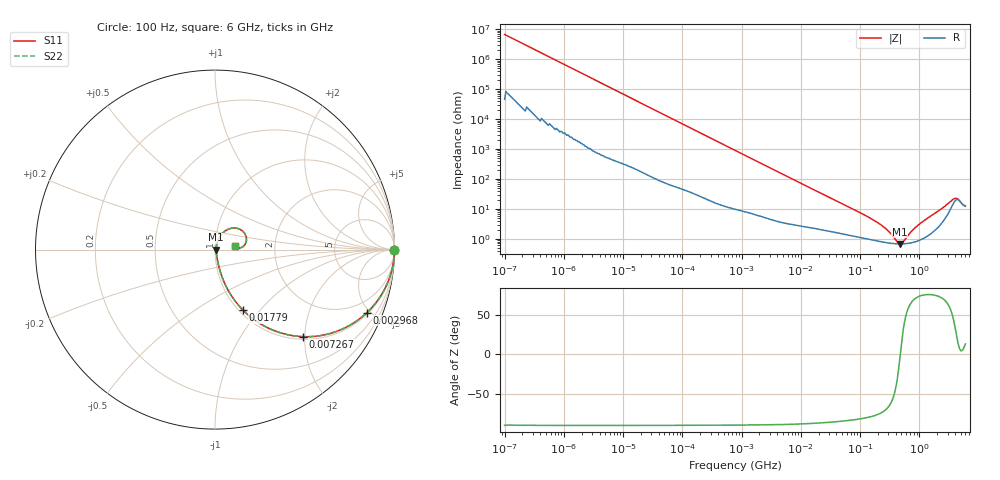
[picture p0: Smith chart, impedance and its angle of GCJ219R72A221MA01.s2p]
!Murata Part Number: GCJ219R72A221MA01
!These Parameters are Measured in Series Mode Connection
!Data Generated on Mar 13, 2026
!  o--ll--o
!Port1  Port2
!  o------o
!Operation Temp=25[degC], DC Bias Voltage=0[V]
!Freq. Start=100[Hz] Stop=6[GHz] 401[Steps]
# Hz S RI R 50
!Freq.(Hz) S11(Real) S11(Imag) S21(Real) S21(Imag) S12(Real) S12(Imag) S22(Real) S22(Imag)
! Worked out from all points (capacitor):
!   401 points, 100 Hz to 6 GHz, reference 50 ohm
!   read as one part in series: C = 234 pF near 109 Hz
!   lowest |Z| = 677 mohm at 467.5 MHz (marker M1)
!   series resonance near 477.6 MHz, so ESL is about 480 pH
!   S11 on the Smith chart (normalised r, x): 100 Hz: open; 2.968 MHz: 1.09, -4.78; 7.267 MHz: 1.06, -1.97; 17.79 MHz: 1.04, -0.81; 6 GHz: 1.25, +0.06
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100  1 -1.47e-05  1e-07 1.47e-05  1e-07 1.47e-05  1 -1.47e-05
656  1 -9.56e-05  5e-07 9.56e-05  5e-07 9.56e-05  1 -9.56e-05
2008  1 -0.000292  1.4e-06 0.000292  1.4e-06 0.000292  1 -0.000292
40335  0.9999 -0.00581  6.39e-05 0.00581  6.39e-05 0.00581  0.9999 -0.00581
774597  0.9868 -0.1088  0.0132 0.1088  0.0132 0.1088  0.9868 -0.1088
1658239  0.9446 -0.2212  0.0554 0.2212  0.0554 0.2212  0.9446 -0.2212
2967816  0.8463 -0.3514  0.1537 0.3514  0.1537 0.3514  0.8463 -0.3514
7266822  0.4917 -0.4851  0.5083 0.4851  0.5083 0.4851  0.4917 -0.4851
1.555665e7  0.1893 -0.3679  0.8107 0.3679  0.8107 0.3679  0.1893 -0.3679
1.779312e7  0.1553 -0.3364  0.8447 0.3364  0.8447 0.3364  0.1553 -0.3364
3.80911e7  0.0504 -0.1806  0.9496 0.1806  0.9496 0.1806  0.0504 -0.1806
1.334425e8  0.0126 -0.0531  0.9874 0.0531  0.9874 0.0531  0.0126 -0.0531
2.183701e8  0.00885 -0.0288  0.9912 0.0288  0.9912 0.0288  0.00885 -0.0288
3.124326e8  0.00734 -0.0149  0.9927 0.0149  0.9927 0.0149  0.00734 -0.0149
4.674818e8  0.00668 -0.000741  0.9933 0.000741  0.9933 0.000741  0.00668 -0.000741
5.346885e8  0.00673 0.00397  0.9933 -0.00397  0.9933 -0.00397  0.00673 0.00397
7.31507e8  0.0075 0.0155  0.9925 -0.0155  0.9925 -0.0155  0.0075 0.0155
1.000774e9  0.00961 0.0289  0.9904 -0.0289  0.9904 -0.0289  0.00961 0.0289
2.34314e9  0.0387 0.0878  0.9613 -0.0878  0.9613 -0.0878  0.0387 0.0878
3.505958e9  0.1193 0.1194  0.8807 -0.1194  0.8807 -0.1194  0.1193 0.1194
4.193612e9  0.1748 0.0691  0.8252 -0.0691  0.8252 -0.0691  0.1748 0.0691
6e9  0.1099 0.0224  0.8901 -0.0224  0.8901 -0.0224  0.1099 0.0224
